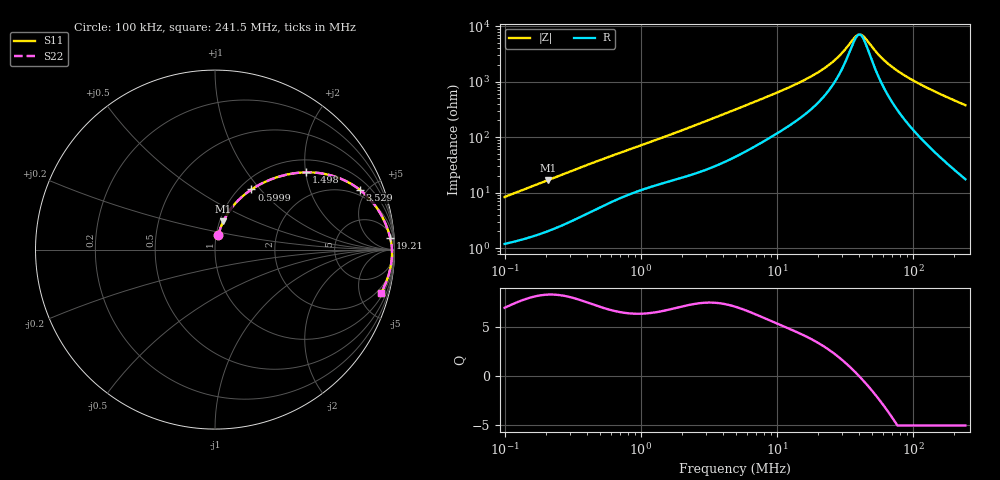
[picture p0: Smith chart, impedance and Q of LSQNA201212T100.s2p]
! LSQNA201212T100  S-PARAMETER MODEL  ( General Type )
! Model Generated by TAIYO YUDEN Corporation (http://www.ty-top.com)
! Version 2.0
! TAIYO YUDEN Control No. 100810NF25SB-FKC
! Copyright(c) 2007 TAIYO YUDEN CO.,LTD. All Rights Reserved.
! Product Description (link to TY-COMPAS)
! https://ds.yuden.co.jp/TYCOMPAS/or/detail?pn=LSQNA201212T100K&u=M
! Products Name : Inductors
! Characteristics :
!  Inductance : 10 uH , SRF(min) : 32 MHz , DC Resistance(max) : 0.91 Ohm
!  Rated Current : Saturation :190 mA , Temp Rise : 440 mA (40 degC)
!  Case Size : 2.0 x 1.25 / 0.079 x 0.049 [mm/inch] , Thickness : 1.25 / 0.049 [mm/inch]
!  (Conditions: Temperature = 25 degC , DC Bias Current/Voltage = 0A / 0V)
! External Node Assignments :
!  1  o---GGG---o  2
! GND o---------o GND
! Frequency Range : 0.1MHz  -  241.513628MHz  [ 402 STEP ]
# MHz S RI R 50
! Freq[MHz].  S11 Real  S11 Imag  S21 Real  S21 Imag  S12 Real  S12 Imag  S22 Real  S22 Imag
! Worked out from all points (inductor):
!   401 points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, 100 kHz to 241.5 MHz, reference 50 ohm
!   read as one part in series: L = 13 uH near 104 kHz
!   highest Q = 8.28 at 209.6 kHz (marker M1), where L = 12.8 uH
!   self-resonance near 40.12 MHz
!   S11 on the Smith chart (normalised r, x): 100 kHz: 1.02, +0.17; 599.9 kHz: 1.13, +0.90; 1.498 MHz: 1.30, +2.01; 3.529 MHz: 1.60, +4.50; 19.21 MHz: 9, +27; 241.5 MHz: 1.35, -7.52
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0.1  0.0184 0.0803  0.9816 -0.0803  0.9816 -0.0803  0.0184 0.0803
0.209594  0.0461 0.1578  0.9539 -0.1578  0.9539 -0.1578  0.0461 0.1578
0.368674  0.1052 0.2484  0.8948 -0.2484  0.8948 -0.2484  0.1052 0.2484
0.599897  0.2033 0.3349  0.7967 -0.3349  0.7967 -0.3349  0.2033 0.3349
1.359207  0.4697 0.4285  0.5303 -0.4285  0.5303 -0.4285  0.4697 0.4285
1.498208  0.5076 0.4305  0.4924 -0.4305  0.4924 -0.4305  0.5076 0.4305
2.211665  0.6588 0.4098  0.3412 -0.4098  0.3412 -0.4098  0.6588 0.4098
3.529359  0.8071 0.3331  0.1929 -0.3331  0.1929 -0.3331  0.8071 0.3331
4.914404  0.8766 0.2657  0.1234 -0.2657  0.1234 -0.2657  0.8766 0.2657
10.7094  0.9542 0.1336  0.0458 -0.1336  0.0458 -0.1336  0.9542 0.1336
18.11814  0.9746 0.0725  0.0254 -0.0725  0.0254 -0.0725  0.9746 0.0725
19.20815  0.9761 0.0666  0.0239 -0.0666  0.0239 -0.0666  0.9761 0.0666
26.74611  0.9824 0.0355  0.0176 -0.0355  0.0176 -0.0355  0.9824 0.0355
30.65223  0.9841 0.0234  0.0159 -0.0234  0.0159 -0.0234  0.9841 0.0234
37.24223  0.9857 0.00646  0.0143 -0.00646  0.0143 -0.00646  0.9857 0.00646
40.25919  0.9861 -0.000302  0.0139 0.000302  0.0139 0.000302  0.9861 -0.000302
43.52056  0.9863 -0.0071  0.0137 0.0071  0.0137 0.0071  0.9863 -0.0071
54.97721  0.9863 -0.0281  0.0137 0.0281  0.0137 0.0281  0.9863 -0.0281
66.79689  0.9853 -0.0467  0.0147 0.0467  0.0147 0.0467  0.9853 -0.0467
84.38097  0.9826 -0.0714  0.0174 0.0714  0.0174 0.0714  0.9826 -0.0714
110.8275  0.9767 -0.1049  0.0233 0.1049  0.0233 0.1049  0.9767 -0.1049
241.5136  0.9243 -0.2424  0.0757 0.2424  0.0757 0.2424  0.9243 -0.2424
